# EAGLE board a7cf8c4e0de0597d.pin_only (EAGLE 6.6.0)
REV: B

Size 36.1 x 22.86 mm. Coordinates in mm from the lower left corner, seen from the top.
Outline: 34.29,22.86 2.54,22.86 arc90 0,20.32 0,15.49 0.25,15.24 0.25,7.62 0,7.37 0,2.54 arc90 2.54,0 34.29,0 arc90 36.07,2.54 36.07,20.32 arc90 34.29,22.86
Copper layers (1*16): Top 0.035mm / dielectric 1.5mm / Bottom 0.035mm
Design rules "adafruit *": minimum track width 8mil, minimum drill 15.5mil, track to track 8mil, track to pad 8mil, pad to pad 8mil, via to via 8mil, smd to smd 8mil, copper to edge 10mil, drill to drill 8mil, minimum pad ring 10mil, minimum via ring 8mil, stop-mask expansion 2mil, vias tented up to drill 20mil, thermal gap 10mil
tRestrict: area 22.9,7.9 to 23.1,8.3; area 24.9,12.1 to 25,12.4; area 24.3,12.1 to 24.4,12.4

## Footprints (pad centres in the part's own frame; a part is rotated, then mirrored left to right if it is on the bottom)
JSTPH2 = smd 1 x 4.6: 1 -1,-3.7; 2 1,-3.7 | smd 1.6 x 3.4: NC1 -3.4,1.5; NC2 3.4,1.5
0805-NO = smd 1.3 x 1.5: 1 -0.95,0; 2 0.95,0
0805_10MGAP = smd 1.2 x 1.5: 1 -1.05,0; 2 1.05,0
C1210 = smd 1.6 x 2.7: 1 -1.4,0; 2 1.4,0
CHIPLED_0805_NOOUTLINE = smd 1.2 x 1.2: A 0,-1.05; C 0,1.05
USB_HOST-PTH = drill 0.95 long: D+ 1,6.52; D- -1,6.52; GND 3.5,6.52; VBUS -3.5,6.52 | drill 2.3 pad 2.9: S1 -6.57,3.81; S2 6.57,3.81
4UCONN_20329 = smd 1 x 2: BASE@1 -0.75,-2; BASE@2 0.75,-2 | smd 0.4 x 1.35: D+ 0,0.775; D- -0.65,0.775; GND 1.3,0.775; ID 0.65,0.775; VBUS -1.3,0.775 | drill 0.7 offset: SPRT@1 -3.3,0.9; SPRT@2 3.3,0.9 | drill 0.6 pad 2.5 square: SPRT@3 -3.6,-1.9; SPRT@4 3.6,-1.9 | hole 0.7: -1.95,0; 1.95,0
FIDUCIAL_1MM = smd 1 x 1: 1 0,0
1X08_ROUND = drill 1 pad 1.676: 1 -8.89,0; 2 -6.35,0; 3 -3.81,0; 4 -1.27,0; 5 1.27,0; 6 3.81,0; 7 6.35,0; 8 8.89,0
INDUCTOR_5X5MM_TDK_VLC5045 = smd 2 x 5: P$1 -1.6,0; P$2 1.6,0
_0805MP = smd 1.2 x 1.3: 1 -1.016,0; 2 1.016,0
SC59-BEC = smd 1 x 1.4: B -0.95,-1.2; C 0,1.2; E 0.95,-1.2
PVQFN-16 = smd 1.05 x 0.35: 1 -2.1,0.975; 2 -2.1,0.325; 3 -2.1,-0.325; 4 -2.1,-0.975; 9 2.1,-0.975; 10 2.1,-0.325; 11 2.1,0.325; 12 2.1,0.975 | smd 0.35 x 1.05: 5 -0.975,-2.1; 6 -0.325,-2.1; 7 0.325,-2.1; 8 0.975,-2.1; 13 0.975,2.1; 14 0.325,2.1; 15 -0.325,2.1; 16 -0.975,2.1 | drill 0.4: P$18 0,0; P$19 -0.9,0.9; P$20 0.9,0.9; P$21 0.9,-0.9; P$22 -0.9,-0.9 | smd 2.7 x 2.7: THERMAL 0,0
QFN20_4MM = smd 0.73 x 0.28: P$1 -1.965,1; P$2 -1.965,0.5; P$3 -1.965,0; P$4 -1.965,-0.5; P$5 -1.965,-1; P$11 1.965,-1; P$12 1.965,-0.5; P$13 1.965,0; P$14 1.965,0.5; P$15 1.965,1 | smd 0.28 x 0.73: P$6 -1,-1.965; P$7 -0.5,-1.965; P$8 0,-1.965; P$9 0.5,-1.965; P$10 1,-1.965; P$16 1,1.965; P$17 0.5,1.965; P$18 0,1.965; P$19 -0.5,1.965; P$20 -1,1.965 | smd 2.5 x 2.5: P$21 0,0
MOUNTINGHOLE_2.5_PLATED = drill 2.5 pad 3.2: P$1 0,0
TERMBLOCK_1X2-3.5MM = drill 1 pad 2.184: 1 1.8,0; 2 -1.7,0

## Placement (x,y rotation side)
B1  JST 2-PH  [JSTPH2]  10.67,19.3 0 top
C1  10uF  [0805-NO]  19.56,16.51 180 top
C2  2.2uF  [0805-NO]  28.45,17.14 270 top
C4  0.1uF  [0805_10MGAP]  19.05,4.45 0 top
C6  100uF  [C1210]  26.16,5.08 270 top
C7  10uF  [0805-NO]  14.22,13.84 0 top
C8  10uF  [0805-NO]  7.11,12.95 90 top
CHRG/LBO  ORANGE  [CHIPLED_0805_NOOUTLINE]  9.78,1.14 270 top
CN1  USBA_FEMALE  [USB_HOST-PTH]  37.72,11.75 90 top
CN4  MicroUSB  [4UCONN_20329]  4.32,11.43 270 top
DONE  GREEN  [CHIPLED_0805_NOOUTLINE]  6.22,1.14 90 top
FID1  FIDUCIAL""  [FIDUCIAL_1MM]  35.18,11.81 0 top
FID2  FIDUCIAL""  [FIDUCIAL_1MM]  10.69,20.34 90 top
FID3  FIDUCIAL""  [FIDUCIAL_1MM]  1.27,5.46 0 top
JP2  [1X08_ROUND]  21.72,1.27 0 top
L1  6.8uH  [INDUCTOR_5X5MM_TDK_VLC5045]  24.4,15.9 0 top
LED1  RED  [CHIPLED_0805_NOOUTLINE]  5.43,20.86 0 top
LED2  BLUE  [CHIPLED_0805_NOOUTLINE]  33.72,1.56 270 top
R1  1.87M  [_0805MP]  19.56,14.61 180 top
R2  340K  [_0805MP]  19.56,12.7 0 top
R3  1.87M  [0805-NO]  23.5,5.59 270 top
R4  200K  [0805-NO]  21.72,6.1 90 top
R5  1K  [0805-NO]  28.7,6.1 270 top
R6  270K  [0805-NO]  15.37,9.65 270 top
R7  100K  [0805-NO]  17.27,9.65 270 top
R8  1K  [0805-NO]  7.49,5.08 270 top
R9  43K  [0805-NO]  28.5,9.91 270 top
R10  49.9K  [0805-NO]  28.48,13.52 90 top
R11  75K 1%  [0805-NO]  29.97,20.57 180 top
R12  49.9K 1%  [0805-NO]  33.4,21.21 0 top
R13  200K  [0805-NO]  19.14,8.89 90 top
R14  1K  [0805-NO]  5.59,4.32 270 top
R16  1.0K  [0805-NO]  12.57,5.08 90 top
R17  100K  [0805-NO]  10.67,5.08 90 top
R20  1K  [0805-NO]  15.84,16.62 270 top
T1  MMUN2133LT1G  [SC59-BEC]  15.7,5.33 0 top
THERM  15K  [0805-NO]  6.99,9.4 90 top
U1  TPS61090RSAR  [PVQFN-16]  24.27,10.21 180 top
U2  MCP73871  [QFN20_4MM]  11.81,9.4 270 top
U$10  MOUNTINGHOLE2.5  [MOUNTINGHOLE_2.5_PLATED]  2.54,20.32 0 top
U$11  MOUNTINGHOLE2.5  [MOUNTINGHOLE_2.5_PLATED]  2.54,2.54 0 top
U$12  [PCBFEAT-REV-040]  11.3,19.56 0 bottom
U$25  [SYMBOL_PLUS]  31.11,6.22 0 top
U$26  [SYMBOL_MINUS]  31.11,17.4 90 top
U$28  [ADAFRUIT_5MM]  6.75,0.58 90 bottom
U$45  [ADAFRUIT_3.5MM]  16.51,17.65 0 top
X1  [TERMBLOCK_1X2-3.5MM]  33.91,11.75 90 top

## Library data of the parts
B1 C1 C2 C4 C7 C8 CHRG/LBO CN1 CN4 DONE JP2 L1 LED1 LED2 R1-R14 R16 R17 R20 THERM U1 U2 U$12 U$25 U$26 U$28 U$45 X1 = microbuilder
C6 = rcl
FID1 FID3 = microbuilder; BOM: EXCLUDE; COMPANY: ADAFRUIT INDUSTRIES; DRAWN: KTOWN; REV: A
FID2 U$10 U$11 = microbuilder; BOM: EXCLUDE
T1 = transistor

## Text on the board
tPlace: PowerBoost 1000C | adafruit | LOW | - | + | PWR | chrg | USB | Bat | Vs | EN | GND | G | 5V
bPlace: PowerBoost 1000 Charger | TPS61090 DC Boost | 5Vout: ~5.2V @ 1A+ output | 3.2V Low Batt Indicator | LiPoly: 3.7V/4.2V Li only! | Vsh: larger of USB/LiPo | USB: 1A Charge Rate | iOS 1A Charge Resistors | USB | LiPo | Vsh | EN | GND | LBO | GND | 5Vo

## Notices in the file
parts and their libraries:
microbuilder: This work is placed in the public domain, and may be freely used for commercial and non-commercial work with the following conditions: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
